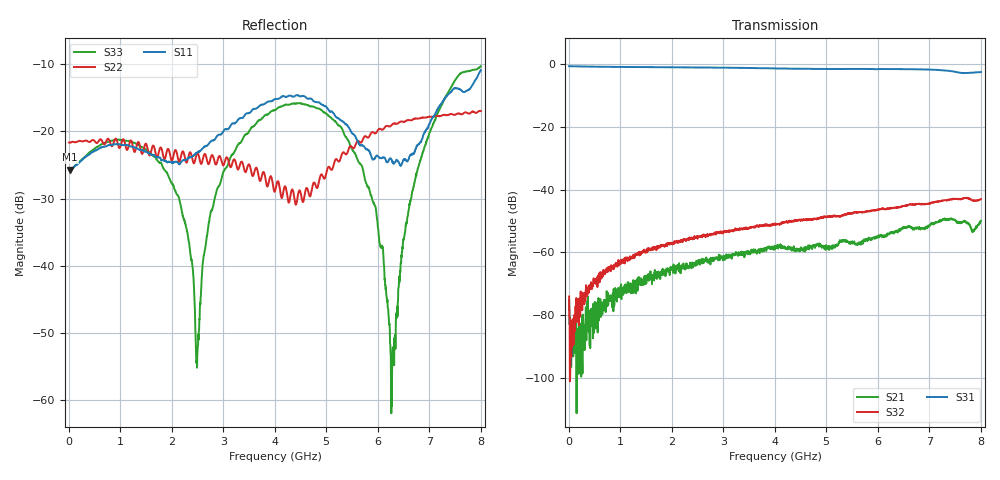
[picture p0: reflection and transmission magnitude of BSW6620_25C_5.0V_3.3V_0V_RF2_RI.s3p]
! Product: BSW6620
! Temp: 25C
! VDD: 5.000
! Control_Hi: 3.300
! Control_Lo: 0.000
! Logic State: RF2
! Port 1: RFC
! Port 2: RF1
! Port 3: RF2
! V1 = 5.00
! V2 = 3.30
! V3 = 0.00
! V4 = 0.00
# Hz S  RI  R 50
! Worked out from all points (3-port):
!   1601 points, 5 MHz to 8.005 GHz, reference 50 ohm
!   strongest paths, dB at 5 MHz, 2.005 GHz, 4.005 GHz, 6.005 GHz, 8.005 GHz:
!     S31: -0.6, -1.0, -1.3, -1.6, -2.5
!     S32: -74.1, -56.9, -51.2, -46.5, -43.0
!     S21: -75.2, -65.2, -58.7, -55.3, -49.9
!   lowest |S11| = -25.7 dB at 25 MHz (marker M1), VSWR 1.11, Z = 55.5 - j0.0595 ohm
!   |S11| at or under -10 dB: start of sweep to end of sweep
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5000000  0.0525 0.000191  0.000149 -0.000121  0.9321 -0.0127
         0.000129 -0.000117  0.0826 -0.00107  0.000177 -0.000102
         0.9322 -0.0132  0.000183 -7.52e-05  0.0522 -5.92e-05
2.5e7  0.0518 -0.000535  3.51e-06 1.93e-05  0.9305 -0.0538
       3.3e-05 -8.49e-05  0.0824 -0.00309  -3.72e-06 -4.49e-05
       0.9308 -0.0506  -1.05e-05 1.49e-06  0.0517 0.00177
7.35e8  0.056 -0.054  0.000111 5.24e-05  0.0299 -0.9104
        0.000207 0.000123  0.0479 -0.0713  0.000541 9.54e-05
        0.0301 -0.9104  0.000546 0.000129  0.0621 -0.055
1.45e9  -0.0447 -0.0559  0.000196 -0.000245  -0.8946 -0.1084
        0.000224 -0.000287  -0.0373 -0.0618  0.00046 -0.00085
        -0.8948 -0.1084  0.000453 -0.000904  -0.0333 -0.0674
2.495e9  0.0462 0.052  -0.000619 -9.3e-05  0.4096 0.7892
         -0.000682 -0.000145  -0.0507 0.0465  -0.00173 -0.000157
         0.4097 0.789  -0.00167 -0.000217  -0.00138 -0.00169
4.005e9  -0.173 0.0165  0.00109 0.000436  -0.3947 -0.7621
         0.00109 0.000409  0.0335 -0.0129  0.00246 0.00126
         -0.3944 -0.7617  0.00243 0.00129  -0.1285 0.0652
5.245e9  0.1073 0.062  -0.000194 -0.00135  -0.0806 0.8339
         -9.32e-05 -0.00147  -0.0565 0.0189  -0.000855 -0.00359
         -0.0806 0.8335  -0.000782 -0.00369  0.0936 0.0585
6.29e9  0.0333 -0.0496  -0.00194 0.000836  0.722 -0.4268
        -0.00185 0.000845  0.0373 0.107  -0.00437 0.00258
        0.7234 -0.4277  -0.00446 0.00252  0.00133 0.00192
6.785e9  -0.0731 -0.0325  -9.16e-05 0.0024  -0.0268 -0.8274
         -7.41e-05 0.00246  0.1044 0.0673  -0.000514 0.00587
         -0.0263 -0.8279  -0.000494 0.00594  -0.0482 0.0227
8.005e9  0.2642 0.1078  0.00187 -0.00254  -0.3826 0.6436
         0.00177 -0.00264  0.0611 -0.1275  0.00519 -0.00475
         -0.3824 0.6444  0.00511 -0.00489  0.2719 0.1382
